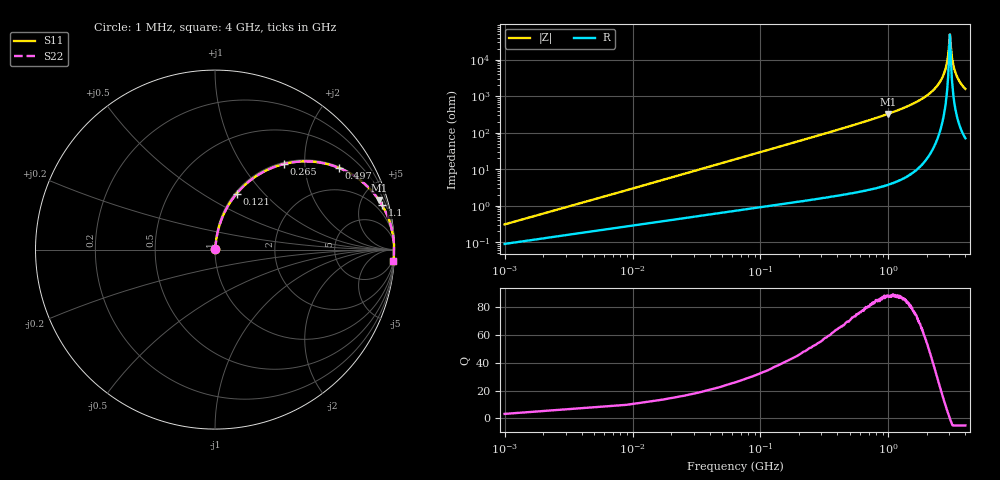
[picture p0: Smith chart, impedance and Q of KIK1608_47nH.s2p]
!version-2
!date-01.2022
!Series
# MHz S RI R 50
!Freq ReS11 ImS11 ReS21 ImS21 ReS12 ImS12 ReS22 ImS22
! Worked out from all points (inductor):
!   501 points, 1 MHz to 4 GHz, reference 50 ohm
!   read as one part in series: L = 47 nH near 17 MHz
!   highest Q = 87.8 at 993 MHz (marker M1), where L = 52.7 nH
!   self-resonance near 3.02 GHz
!   S11 on the Smith chart (normalised r, x): 1 MHz: 1.00, +0.01; 121 MHz: 1.02, +0.72; 265 MHz: 1.03, +1.58; 497 MHz: 1.04, +3.02; 1.1 GHz: 1.09, +7.53; 4 GHz: 2, -32
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1  0.000916 0.00295  0.9991 -0.00295  0.9991 -0.00295  0.000916 0.00295
25  0.00987 0.0728  0.9901 -0.0728  0.9901 -0.0728  0.00987 0.0728
33  0.0145 0.0956  0.9855 -0.0956  0.9855 -0.0956  0.0145 0.0956
65  0.0421 0.1826  0.9579 -0.1826  0.9579 -0.1826  0.0421 0.1826
121  0.1204 0.3117  0.8796 -0.3117  0.8796 -0.3117  0.1204 0.3117
265  0.3856 0.4773  0.6144 -0.4773  0.6144 -0.4773  0.3856 0.4773
497  0.6922 0.4545  0.3078 -0.4545  0.3078 -0.4545  0.6922 0.4545
673  0.8108 0.3854  0.1892 -0.3854  0.1892 -0.3854  0.8108 0.3854
993  0.9126 0.2768  0.0874 -0.2768  0.0874 -0.2768  0.9126 0.2768
1100  0.9316 0.2467  0.0683 -0.2467  0.0683 -0.2467  0.9316 0.2467
1335  0.958 0.1949  0.042 -0.1949  0.042 -0.1949  0.958 0.1949
2010  0.9895 0.0932  0.0105 -0.0932  0.0105 -0.0932  0.9895 0.0932
2670  0.9974 0.0279  0.0026 -0.0279  0.0026 -0.0279  0.9974 0.0279
2890  0.998 0.0105  0.00203 -0.0105  0.00203 -0.0105  0.998 0.0105
2970  0.998 0.00443  0.00198 -0.00443  0.00198 -0.00443  0.998 0.00443
3020  0.998 0.000272  0.002 -0.000272  0.002 -0.000272  0.998 0.000272
3050  0.998 -0.00149  0.00201 0.00149  0.00201 0.00149  0.998 -0.00149
3100  0.9979 -0.00554  0.00208 0.00554  0.00208 0.00554  0.9979 -0.00554
3140  0.9979 -0.00839  0.00214 0.00839  0.00214 0.00839  0.9979 -0.00839
3335  0.9973 -0.0216  0.00268 0.0216  0.00268 0.0216  0.9973 -0.0216
3620  0.9959 -0.0401  0.00406 0.0401  0.00406 0.0401  0.9959 -0.0401
4000  0.9933 -0.0624  0.00673 0.0624  0.00673 0.0624  0.9933 -0.0624
